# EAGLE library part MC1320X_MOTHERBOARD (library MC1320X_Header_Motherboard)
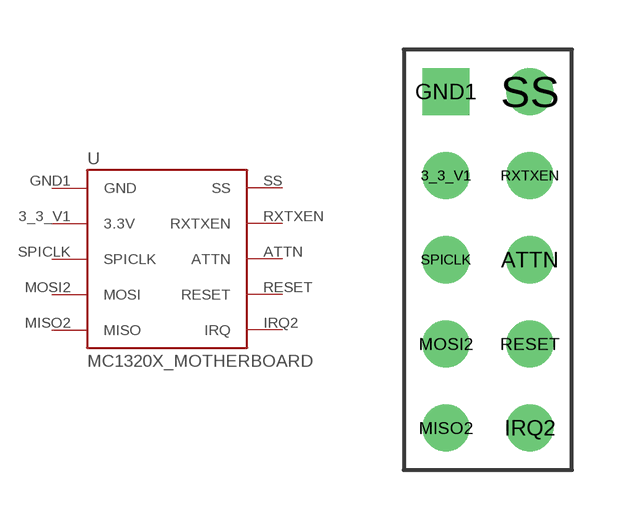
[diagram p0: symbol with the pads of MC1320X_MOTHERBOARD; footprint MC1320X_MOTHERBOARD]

Designator prefix -

## MC1320X_MOTHERBOARD  [MC1320X_MOTHERBOARD]
3_3_V1  3.3V
ATTN  ATTN
GND1  GND
IRQ2  IRQ
MISO2  MISO
MOSI2  MOSI
RESET  RESET
RXTXEN  RXTXEN
SPICLK  SPICLK
SS  SS

## Footprint MC1320X_MOTHERBOARD (pad centres in mm)
drill 0.9 pad 1.422: 3_3_V1 -1.27,3.81; ATTN 1.27,1.27; IRQ2 1.27,-3.81; MISO2 -1.27,-3.81; MOSI2 -1.27,-1.27; RESET 1.27,-1.27; RXTXEN 1.27,3.81; SPICLK -1.27,1.27; SS 1.27,6.35
drill 0.9 pad 1.422 square: GND1 -1.27,6.35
